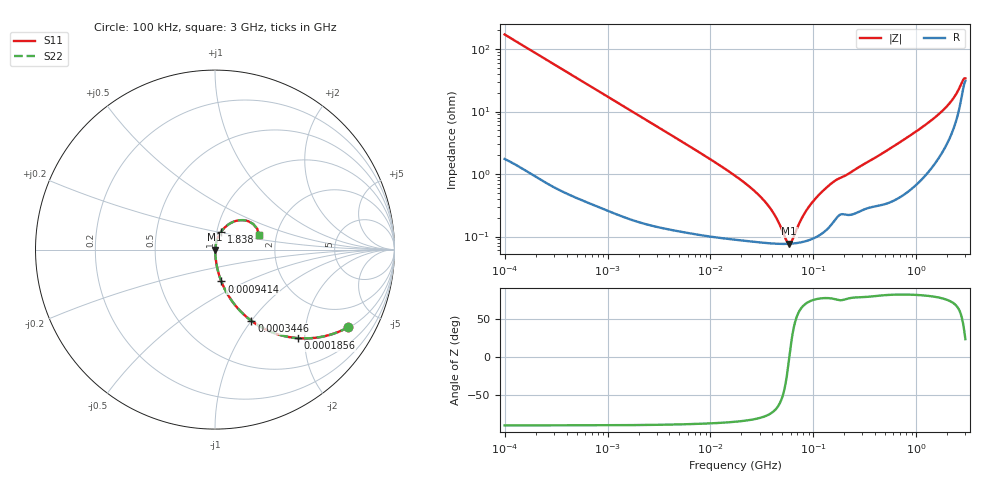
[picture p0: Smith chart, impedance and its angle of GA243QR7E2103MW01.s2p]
!Murata Part Number: GA243QR7E2103MW01
!These Parameters are Measured in Series Mode Connection
!Data Generated on Jun 19, 2026
!  o--ll--o
!Port1  Port2
!  o------o
!Operation Temp=25[degC], DC Bias Voltage=0[V]
!Freq. Start=100[kHz] Stop=3[GHz] 401[Steps]
# Hz S RI R 50
!Freq.(Hz) S11(Real) S11(Imag) S21(Real) S21(Imag) S12(Real) S12(Imag) S22(Real) S22(Imag)
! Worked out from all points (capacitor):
!   401 points, 100 kHz to 3 GHz, reference 50 ohm
!   read as one part in series: C = 9.28 nF near 105.3 kHz
!   lowest |Z| = 76.7 mohm at 58.16 MHz (marker M1)
!   series resonance near 58.36 MHz, so ESL is about 800 pH
!   S11 on the Smith chart (normalised r, x): 100 kHz: 1.03, -3.42; 185.6 kHz: 1.02, -1.85; 344.6 kHz: 1.01, -1.00; 941.4 kHz: 1.01, -0.37; 1.838 GHz: 1.05, +0.21; 3 GHz: 1.62, +0.28
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100000  0.7433 -0.4317  0.2567 0.4317  0.2567 0.4317  0.7433 -0.4317
185621  0.4623 -0.4933  0.5377 0.4933  0.5377 0.4933  0.4623 -0.4933
344552  0.2032 -0.3969  0.7968 0.3969  0.7968 0.3969  0.2032 -0.3969
562235  0.0894 -0.2792  0.9106 0.2792  0.9106 0.2792  0.0894 -0.2792
941399  0.0353 -0.1774  0.9647 0.1774  0.9647 0.1774  0.0353 -0.1774
3161081  0.00443 -0.0549  0.9956 0.0549  0.9956 0.0549  0.00443 -0.0549
1.77727e7  0.000968 -0.00909  0.999 0.00909  0.999 0.00909  0.000968 -0.00909
2.684345e7  0.00085 -0.00527  0.9991 0.00527  0.9991 0.00527  0.00085 -0.00527
3.564176e7  0.000796 -0.00318  0.9992 0.00318  0.9992 0.00318  0.000796 -0.00318
4.268829e7  0.000773 -0.00198  0.9992 0.00198  0.9992 0.00198  0.000773 -0.00198
5.383243e7  0.000763 -0.000506  0.9992 0.000506  0.9992 0.000506  0.000763 -0.000506
5.815973e7  0.000766 -2.11e-05  0.9992 2.11e-05  0.9992 2.11e-05  0.000766 -2.11e-05
6.283488e7  0.000773 0.000465  0.9992 -0.000465  0.9992 -0.000465  0.000773 0.000465
8.130716e7  0.000835 0.00213  0.9992 -0.00213  0.9992 -0.00213  0.000835 0.00213
9.738194e7  0.000928 0.00339  0.9991 -0.00339  0.9991 -0.00339  0.000928 0.00339
1.589065e8  0.00182 0.00741  0.9982 -0.00741  0.9982 -0.00741  0.00182 0.00741
5.475153e8  0.0041 0.0248  0.9959 -0.0248  0.9959 -0.0248  0.0041 0.0248
1.156079e9  0.0116 0.0554  0.9884 -0.0554  0.9884 -0.0554  0.0116 0.0554
1.838476e9  0.0335 0.0983  0.9665 -0.0983  0.9665 -0.0983  0.0335 0.0983
2.318426e9  0.073 0.1387  0.927 -0.1387  0.927 -0.1387  0.073 0.1387
2.637286e9  0.1367 0.1639  0.8633 -0.1639  0.8633 -0.1639  0.1367 0.1639
3e9  0.2452 0.0793  0.7548 -0.0793  0.7548 -0.0793  0.2452 0.0793
